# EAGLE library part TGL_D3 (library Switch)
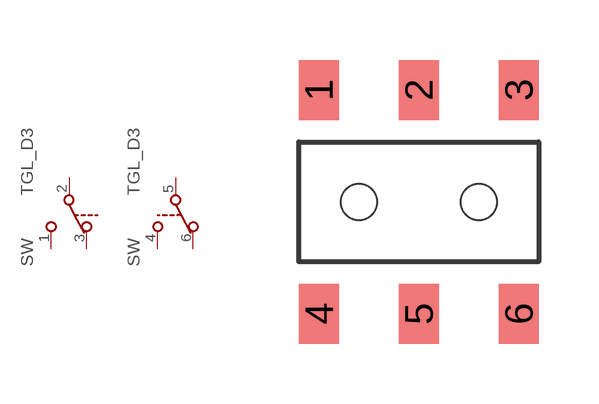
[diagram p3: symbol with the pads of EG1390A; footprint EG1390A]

Designator prefix SW; gates G$1=TGL_3- G$2=TGL_-3

## TGL_D3EG1390  [EG1390A]
1  G$1:1  pas
2  G$1:2  pas
3  G$1:3  pas
4  G$2:1  pas
5  G$2:2  pas
6  G$2:3  pas

## Footprint EG1390A (pad centres in mm)
EG1390 Producted by E SWITCH Store Information : Digi-Key :
smd 1 x 1.5: 1 -2.5,2.8; 2 0,2.8; 3 2.5,2.8; 4 -2.5,-2.8; 5 0,-2.8; 6 2.5,-2.8
hole 0.9 at -1.5,0
hole 0.9 at 1.5,0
